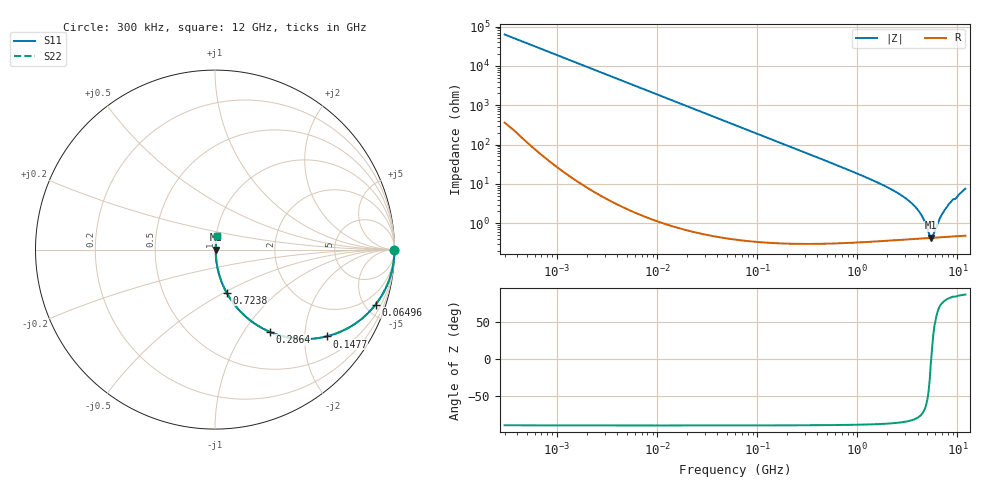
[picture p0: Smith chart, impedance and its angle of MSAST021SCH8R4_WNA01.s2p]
! MSAST021SCH8R4_WNA01  S-PARAMETER MODEL  ( General Type )
! Model Generated by TAIYO YUDEN Corporation (http://www.ty-top.com)
! Version 2.0
! TAIYO YUDEN Control No. 181101
! Copyright(c) 2015 TAIYO YUDEN CO.,LTD. All Rights Reserved.
! Product Description (link to TY-COMPAS)
! https://ds.yuden.co.jp/TYCOMPAS/or/detail?pn=MSAST021SCH8R4CWNA01&u=M
! Products Name : Multilayer Ceramic Capacitors
! Characteristics :
!  Capacitance : 8.4 pF , Rated Voltage : 25V , TCC : CH / C0H
!  Case Size : 0.25 x 0.125 / 0.0098 x 0.0049 [mm/inch] , Thickness : 0.125 / 0.0049 [mm/inch]
!  (Conditions: Temperature = 25 degC , DC Bias Current/Voltage = 0A / 0V)
! External Node Assignments :
!  1  o---| |---o  2
! GND o---------o GND
! Frequency Range : 0.3MHz  -  12000MHz  [ 401 STEP ]
# MHz S RI R 50
! Freq[MHz].  S11 Real  S11 Imag  S21 Real  S21 Imag  S12 Real  S12 Imag  S22 Real  S22 Imag
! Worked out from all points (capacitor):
!   401 points, 300 kHz to 12 GHz, reference 50 ohm
!   read as one part in series: C = 8.4 pF near 316.3 kHz
!   lowest |Z| = 430 mohm at 5.42 GHz (marker M1)
!   series resonance near 5.472 GHz, so ESL is about 100 pH
!   S11 on the Smith chart (normalised r, x): 300 kHz: open; 64.96 MHz: 1.01, -5.83; 147.7 MHz: 1.01, -2.56; 286.4 MHz: 1.01, -1.32; 723.8 MHz: 1.01, -0.51; 12 GHz: 1.01, +0.15
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0.3  1 -0.00158  1.16e-05 0.00158  1.16e-05 0.00158  1 -0.00158
1.769972  0.9999 -0.00934  9.58e-05 0.00934  9.58e-05 0.00934  0.9999 -0.00934
10.44266  0.9969 -0.0549  0.00306 0.0549  0.00306 0.0549  0.9969 -0.0549
27.10171  0.9798 -0.1401  0.0202 0.1401  0.0202 0.1401  0.9798 -0.1401
60  0.9086 -0.2876  0.0914 0.2876  0.0914 0.2876  0.9086 -0.2876
64.96309  0.8945 -0.3066  0.1055 0.3066  0.1055 0.3066  0.8945 -0.3066
96.65937  0.793 -0.4043  0.207 0.4043  0.207 0.4043  0.793 -0.4043
147.6816  0.6214 -0.4838  0.3786 0.4838  0.3786 0.4838  0.6214 -0.4838
286.3882  0.3041 -0.4578  0.6959 0.4578  0.6959 0.4578  0.3041 -0.4578
353.9943  0.2225 -0.4131  0.7775 0.4131  0.7775 0.4131  0.2225 -0.4131
723.8279  0.0646 -0.2398  0.9354 0.2398  0.9354 0.2398  0.0646 -0.2398
2088.533  0.00951 -0.0764  0.9905 0.0764  0.9905 0.0764  0.00951 -0.0764
3026.31  0.0057 -0.043  0.9943 0.043  0.9943 0.043  0.0057 -0.043
3841.137  0.00462 -0.0247  0.9954 0.0247  0.9954 0.0247  0.00462 -0.0247
4502.883  0.0043 -0.0133  0.9957 0.0133  0.9957 0.0133  0.0043 -0.0133
5140.631  0.00423 -0.00414  0.9958 0.00414  0.9958 0.00414  0.00423 -0.00414
5420.343  0.00425 -0.000484  0.9957 0.000484  0.9957 0.000484  0.00425 -0.000484
5715.274  0.0043 0.00251  0.9957 -0.00251  0.9957 -0.00251  0.0043 0.00251
6699.894  0.00457 0.0129  0.9954 -0.0129  0.9954 -0.0129  0.00457 0.0129
7854.144  0.00516 0.0254  0.9948 -0.0254  0.9948 -0.0254  0.00516 0.0254
8732.115  0.00591 0.0362  0.9941 -0.0362  0.9941 -0.0362  0.00591 0.0362
12000  0.0104 0.0744  0.9896 -0.0744  0.9896 -0.0744  0.0104 0.0744
